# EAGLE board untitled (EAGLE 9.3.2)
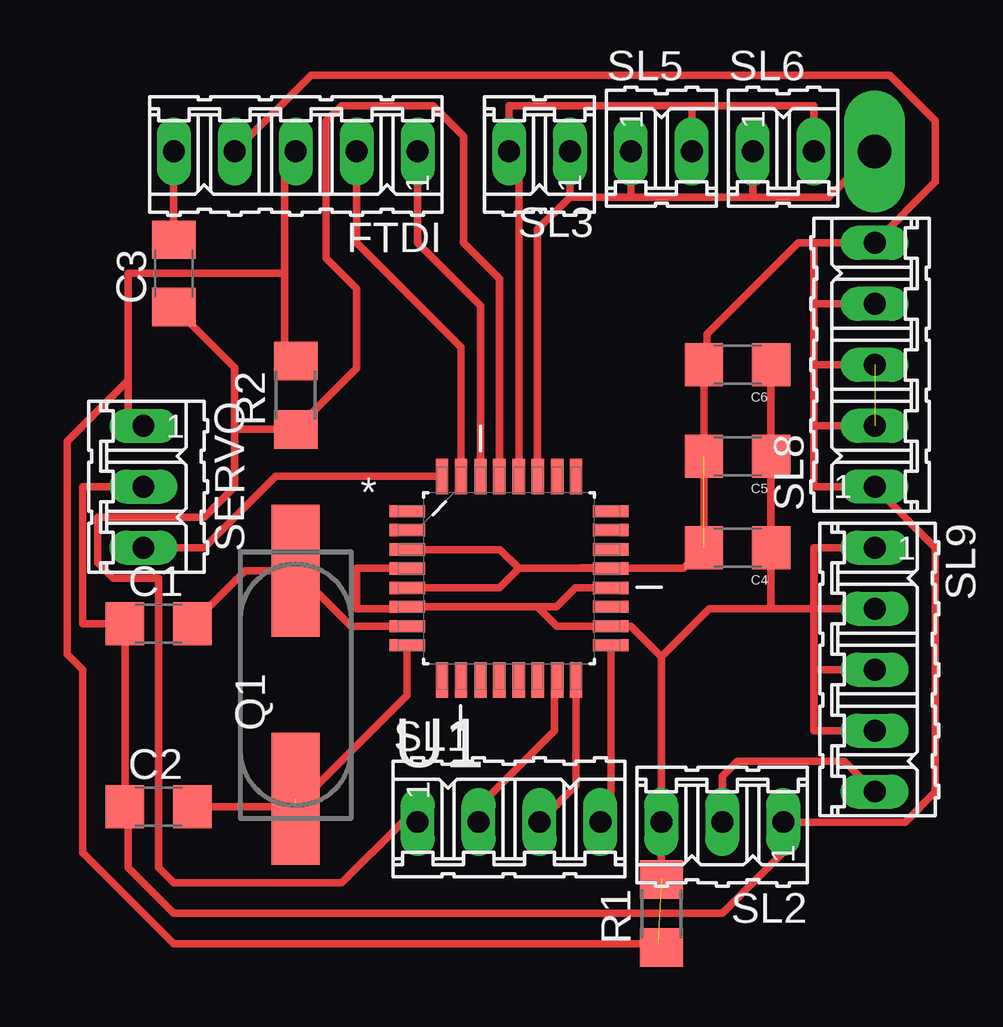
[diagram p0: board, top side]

No outline drawn. Coordinates in mm, seen from the top.
Copper layers (1*16): Top 0.035mm / dielectric 1.5mm / Bottom 0.035mm
Design rules "default": minimum track width 6mil, minimum drill 0.35mm, track to track 6mil, track to pad 6mil, pad to pad 6mil, via to via 6mil, smd to smd 6mil, copper to edge 40mil, drill to drill 6mil, minimum pad ring 10mil, minimum via ring 8mil, stop-mask expansion 4mil, vias tented up to drill 0mil, thermal gap 10mil

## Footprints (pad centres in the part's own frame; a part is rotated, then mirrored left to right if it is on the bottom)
C1206 = smd 1.6 x 1.8: 1 -1.4,0; 2 1.4,0
1206 = smd 1.6 x 1.8: 1 -1.4,0; 2 1.4,0
05P = drill 0.914 long: 1 -5.08,0; 2 -2.54,0; 3 0,0; 4 2.54,0; 5 5.08,0
1X1-BIGPOGO = drill 1.4 pad 2.54 long: P$1 0,0
CSM-7X-DU = smd 5.5 x 2: 1 -4.75,0; 2 4.75,0
R1206 = smd 1.6 x 1.803: 1 -1.422,0; 2 1.422,0
03P = drill 0.914 long: 1 -2.54,0; 2 0,0; 3 2.54,0
04P = drill 0.914 long: 1 -3.81,0; 2 -1.27,0; 3 1.27,0; 4 3.81,0
02P = drill 0.914 long: 1 -1.27,0; 2 1.27,0
QFP80P900X900X120-32N = smd 1.473 x 0.508: 1 -4.242,2.794; 2 -4.242,2.007; 3 -4.242,1.194; 4 -4.242,0.406; 5 -4.242,-0.406; 6 -4.242,-1.194; 7 -4.242,-2.007; 8 -4.242,-2.794; 17 4.242,-2.794; 18 4.242,-2.007; 19 4.242,-1.194; 20 4.242,-0.406; 21 4.242,0.406; 22 4.242,1.194; 23 4.242,2.007; 24 4.242,2.794 | smd 0.508 x 1.473: 9 -2.794,-4.242; 10 -2.007,-4.242; 11 -1.194,-4.242; 12 -0.406,-4.242; 13 0.406,-4.242; 14 1.194,-4.242; 15 2.007,-4.242; 16 2.794,-4.242; 25 2.794,4.242; 26 2.007,4.242; 27 1.194,4.242; 28 0.406,4.242; 29 -0.406,4.242; 30 -1.194,4.242; 31 -2.007,4.242; 32 -2.794,4.242

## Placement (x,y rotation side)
C1  [C1206]  -34.92,-5.71 0 top
C2  [C1206]  -34.92,-13.34 0 top
C3  [C1206]  -34.29,8.89 90 top
C4  10uF  [1206]  -10.79,-2.54 180 top
C5  1uF  [1206]  -10.79,1.27 180 top
C6  100nF  [1206]  -10.79,5.08 180 top
FTDI  [05P]  -29.21,13.97 180 top
JP2  [1X1-BIGPOGO]  -5.08,13.97 90 top
Q1  CSM-7X-DU  [CSM-7X-DU]  -29.21,-8.26 90 top
R1  [R1206]  -13.97,-17.78 90 top
R2  [R1206]  -29.21,3.81 90 top
SERVO  [03P]  -35.56,0 270 top
SL1  [04P]  -20.32,-13.97 0 top
SL2  [03P]  -11.43,-13.97 180 top
SL3  [02P]  -19.05,13.97 180 top
SL5  [02P]  -13.97,13.97 0 top
SL6  [02P]  -8.89,13.97 0 top
SL8  [05P]  -5.08,5.08 90 top
SL9  [05P]  -5.08,-7.62 270 top
U1  ATMEGA328P-AU  [QFP80P900X900X120-32N]  -20.32,-3.81 0 top

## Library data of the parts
C1-C3 JP2 = adafruit
C4-C6 = 01_SparkFun
FTDI SERVO SL1-SL3 SL5 SL6 SL8 SL9 = con-amp-quick; OC_FARNELL: unknown; OC_NEWARK: unknown
Q1 = FAB_Hello; OC_FARNELL: unknown; OC_NEWARK: unknown
R1 R2 = eagle-ltspice; SPICEMODEL: NONE; SPICEPREFIX: R
U1 = Atmel-ATMEGA328P-AU; DESCRIPTION: 8-bit Microcontroller with In-System Programmable Flash; MPN: ATMEGA328P-AU; OC_FARNELL: 1715486; OC_NEWARK: 14R4631; PACKAGE: TQFP-32; SUPPLIER: Atmel

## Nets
GND: C1.1 C2.1 C4.2 C5.2 C6.2 FTDI.4 SERVO.2 SL2.1 SL8.1 SL8.2 SL8.3 SL8.4 SL8.5 U1.3 U1.5 U1.21
MISO: SL1.3 U1.16
MOSI: SL1.2 U1.15
N$1: SL2.2 SL9.5
N$2: C1.2 Q1.2 U1.7
N$3: C2.2 Q1.1 U1.8
RST: C3.1 R2.1 SL1.1 U1.29
RST_FTDI: C3.2 FTDI.5
RX: FTDI.1 U1.30
SCK: SL1.4 U1.17
SCL: SL3.2 SL5.2 SL6.2 U1.28
SDA: JP2.P$1 SL3.1 SL5.1 SL6.1 U1.27
SERV_DATA: SERVO.3 U1.32
TX: FTDI.2 U1.31
VCC: C4.1 C5.1 C6.1 FTDI.3 R1.1 R1.2 R2.2 SERVO.1 SL2.3 SL9.1 SL9.2 SL9.3 SL9.4 U1.4 U1.6 U1.18 U1.20

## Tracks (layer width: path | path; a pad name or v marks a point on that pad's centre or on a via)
GND  (2 unrouted)
  Top 0.305: U1.5 -20.73,-4.22 -19.91,-3.4 | -19.91,-3.4 U1.21 | U1.3 -20.7,-2.62 -19.91,-3.4 | -16.08,-3.38 -17.32,-3.38 -17.3,-3.4 U1.21 | -7.62,2.54 -7.62,0 SL8.1 -2.54,-2.54 -2.54,-12.7 -3.81,-13.97 SL2.1 -8.89,-15.24 -11.43,-17.78 -34.29,-17.78 -36.2,-15.88 -36.2,-13.46 C2.1 C1.1 -38.1,-5.71 -38.1,0 SERVO.2 | -7.62,2.54 -7.62,7.62 | -7.62,7.62 -7.62,10.16 | -7.62,10.16 SL8.5 -2.54,12.7 -2.54,15.24 -4.45,17.14 -28.57,17.14 FTDI.4 | SL8.4 -7.62,7.62 | SL8.3 -7.62,5.08 | SL8.2 -7.62,2.54 | U1.21 -13.06,-3.4 C4.2 C6.2 -12.06,5.21 -12.06,6.35 -8.26,10.16 -7.62,10.16
MISO
  Top 0.305: SL1.3 -17.53,-12.45 U1.16
MOSI
  Top 0.305: U1.15 -18.41,-8.15 -18.41,-10.16 -21.59,-13.34 SL1.2
N$1
  Top 0.305: SL2.2 -11.43,-12.06 -10.79,-11.43 -6.35,-11.43 SL9.5
N$2
  Top 0.305: C1.2 -31.32,-3.5 Q1.2 -26.9,-5.82 U1.7
N$3  (1 unrouted)
  Top 0.305: C2.2 -29.21,-13.34 -24.56,-8.69 U1.8
RST
  Top 0.305: R2.1 -29.06,2.54 | -34.92,6.86 C3.1 -31.75,4.95 -31.75,2.39 | -31.75,2.39 R2.1 | SL1.1 -24.77,-13.97 -27.3,-16.51 -34.29,-16.51 -34.92,-15.88 -34.92,-3.81 -36.83,-3.81 -37.47,-3.17 -37.47,-1.27 -33.02,-1.27 -31.75,0 -31.75,2.39 | U1.29 -20.73,8.66 -22.23,10.16 -22.23,14.61 -23.5,15.88 -27.3,15.88 -27.94,15.24 -27.94,9.53 -26.67,8.26 -26.67,4.93 R2.1
RST_FTDI
  Top 0.305: FTDI.5 C3.2
RX
  Top 0.305: FTDI.1 -24.13,10.16 -21.51,7.54 U1.30
SCK
  Top 0.305: SL1.4 -16.08,-13.54 U1.17
SCL
  Top 0.305: U1.28 -19.91,13.56 SL3.2 -20.32,15.88 -12.7,15.88 | -12.7,15.88 SL5.2 | -12.7,15.88 -7.62,15.88 SL6.2
SDA
  Top 0.305: SL3.1 -17.78,12.06 | U1.27 -19.13,10.72 -17.78,12.06 | SL5.1 -15.24,12.06 | -15.24,12.06 -17.78,12.06 | -15.24,12.06 -10.16,12.06 | -10.16,12.06 SL6.1 | -10.16,12.06 -6.99,12.06 JP2.P$1
SERV_DATA
  Top 0.305: SERVO.3 -33.02,-2.54 -30.05,0.43 U1.32
TX
  Top 0.305: FTDI.2 -26.67,10.16 -22.33,5.82 U1.31
VCC  (1 unrouted)
  Top 0.305: -19.13,-5 U1.6 -24.64,-5.08 -26.67,-5.08 -26.67,-3.4 U1.4 | -19.13,-5 -18.31,-5.82 U1.18 -15.24,-5.82 -13.97,-7.09 | -13.97,-7.09 SL2.3 R1.2 | -9.53,-5.08 -7.62,-5.08 | -7.62,-5.08 SL9.2 | -7.62,-5.08 -7.62,-2.54 SL9.1 | -7.62,-5.08 -7.62,-7.62 | -7.62,-7.62 SL9.3 | -7.62,-7.62 -7.62,-10.16 SL9.4 | FTDI.3 -29.67,13.51 -29.67,8.89 | -29.67,8.89 -29.67,5.69 R2.2 | C6.1 C5.1 C4.1 -9.39,-4.95 -9.53,-5.08 | -19.13,-5 -18.34,-5 -17.55,-4.22 U1.20 | -36.2,4.45 -36.2,8.89 -29.67,8.89 | -36.2,4.45 -36.2,3.17 SERVO.1 | R1.1 -14.12,-19.05 -34.3,-19.05 -38.1,-15.25 -38.1,-7.62 -38.73,-6.99 -38.73,1.91 -36.2,4.45 | -13.97,-7.09 -11.96,-5.08 -9.53,-5.08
